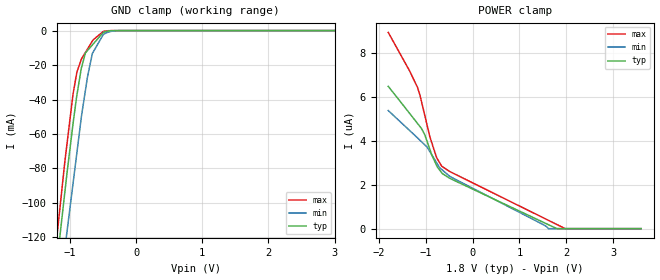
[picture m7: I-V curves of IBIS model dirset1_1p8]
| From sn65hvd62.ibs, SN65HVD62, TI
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|   dirset1_1p8 Model
[Model]   dirset1_1p8
Model_type   Input
Vinl = 0.54
Vinh = 1.26
|   typ   min   max
|   (nom PVT)   (fast PVT)   (slow PVT)
 C_comp   2.168e-12   2.155e-12   2.246e-12
| Where nom  PVT is Nominal Process, 1.8V, 27C
|   Fast PVT is Strong Process,  1.98V, -40C
|   Slow PVT is Weak Process,   1.62V, 125C
[Voltage Range]   1.8   1.62   1.98
|Ambient Temperature   25   85   -40
|Junction Temperature
[Temperature Range]   27   125   -40
[Power Clamp Reference]   1.8   1.62   1.98
[GND Clamp Reference]   0   0   0
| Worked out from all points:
|   GND clamp passes 1 mA (typ) near -0.49 V on its own axis
[GND Clamp]
|   Voltage   I(typ)   I(min)   I(max)
-1.8V     -356.6mA   -371.3mA   -354.8mA
-1.242V   -151mA     -181.4mA   -136.8mA
-1.145V   -118mA     -148.5mA   -101.8mA
-1.042V   -82.82mA   -116.8mA   -65.84mA
-948.4mV  -53.35mA   -88mA      -36.33mA
-893mV    -37.63mA   -70.97mA   -24.21mA
-826.2mV  -21.87mA   -50.46mA   -16.73mA
-763.2mV  -12.93mA   -34.57mA   -12.65mA
-659.3mV  -8.367mA   -13.31mA   -6.076mA
-495mV    -1.153mA   -2.358mA   -544.5uA
-241.4mV  -2.387uA   -29.8uA    -624nA
3.6V      0A         0A         0A
[POWER Clamp]
|   Voltage   I(typ)   I(min)   I(max)
-1.8V     6.465uA    5.366uA    8.916uA
-1.176V   4.784uA    4.128uA    6.422uA
-1.119V   4.628uA    4.009uA    6.033uA
-1.024V   4.288uA    3.814uA    5.187uA
-906.8mV  3.574uA    3.486uA    4.136uA
-762.3mV  2.846uA    2.977uA    3.207uA
-655.4mV  2.531uA    2.682uA    2.833uA
-427.7mV  2.228uA    2.31uA     2.534uA
1.618V    182nA      0A         380.5nA
1.798V    0A         0A         191.3nA
1.978V    0A         0A         0A
3.6V      0A         0A         0A
